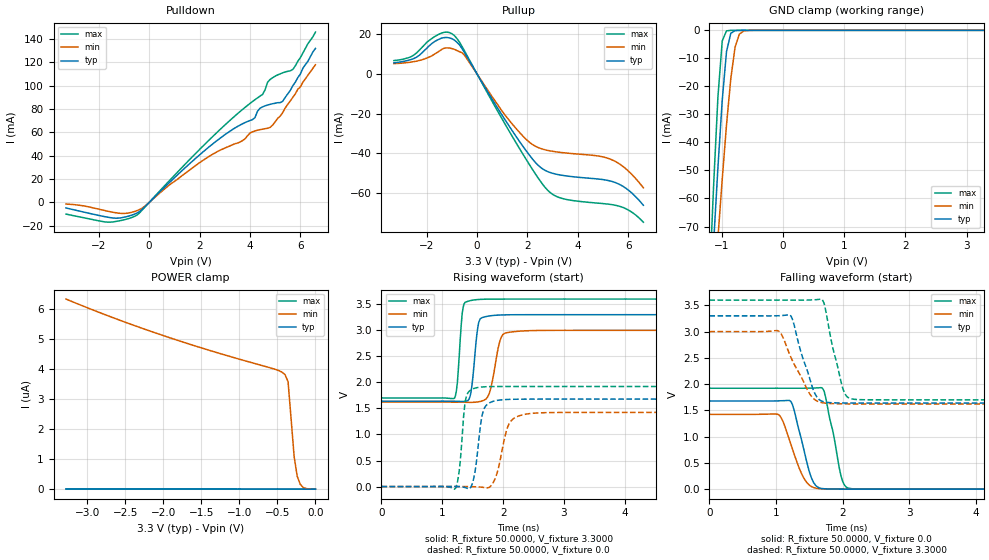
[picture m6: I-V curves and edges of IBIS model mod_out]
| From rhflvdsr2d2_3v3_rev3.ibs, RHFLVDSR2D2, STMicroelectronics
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|   Model mod_out
[Model]   mod_out
Model_type 3-state
Polarity   Non-Inverting
Enable   Active-High
Vmeas  =   1.650V
Cref   =   10pF
C_comp   0.640pF   0.584pF   0.702pF
[Temperature Range]  25.0000   0.1250k   -55.0000
[Voltage Range]   3.3000V   3.0000V   3.6000V
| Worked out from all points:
|   slope of the pulldown table from 0 to 0.495 V, typ, clamps not added: 46.8 ohm
|   slope of the pullup table from 0 to 0.495 V, typ, clamps not added: 46.9 ohm
|   GND clamp passes 1 mA (typ) near -0.85 V on its own axis
|   rising waveform, R_fixture 50.0000, V_fixture 3.3000: 20-80 % time 83.5ps typ, 133ps min, 66.4ps max; typ from 1.64 V to 3.3 V
|   rising waveform, R_fixture 50.0000, V_fixture 0.0: 20-80 % time 106ps typ, 167ps min, 81.1ps max; typ from 0 V to 1.68 V
|   falling waveform, R_fixture 50.0000, V_fixture 0.0: 20-80 % time 196ps typ, 239ps min, 176ps max; typ from 1.68 V to 0 V
|   falling waveform, R_fixture 50.0000, V_fixture 3.3000: 20-80 % time 236ps typ, 313ps min, 197ps max; typ from 3.3 V to 1.64 V
[Pulldown]
|Voltage   I(typ)   I(min)   I(max)
-3.3V     -4.744mA   -1.373mA   -9.997mA
-1.6V     -12.82mA   -7.695mA   -16.93mA
-1V       -12.69mA   -9.437mA   -14.89mA
-500mV    -9.257mA   -7.15mA    -11.05mA
2.4V      47.99mA    39.74mA    53.91mA
3.6V      66.23mA    51.68mA    77.75mA
4.1V      70.95mA    60.5mA     86.46mA
4.5V      81.9mA     62.8mA     92.56mA
4.8V      84.1mA     64.3mA     105.4mA
5.3V      86.7mA     77mA       111.1mA
5.7V      100mA      90mA       114mA
6.6V      132mA      118mA      146mA
[Pullup]
|Voltage   I(typ)   I(min)   I(max)
-3.3V     5.65mA     5.22mA     6.74mA
-2.4V     8.45mA     6.46mA     10.62mA
-1.5V     17.55mA    11.5mA     20.1mA
-1V       17.77mA    12.8mA     20.31mA
-500mV    10.83mA    9.442mA    11.64mA
1V        -20.88mA   -18.83mA   -22.78mA
1.8V      -36.04mA   -31mA      -39.95mA
2.8V      -49.13mA   -38.47mA   -58.51mA
3.5V      -51.26mA   -39.75mA   -63.05mA
5.3V      -53.92mA   -42.94mA   -65.68mA
5.9V      -57.48mA   -47.67mA   -67.81mA
6.6V      -66.12mA   -57.33mA   -74.62mA
[GND_clamp]
|Voltage   I(typ)   I(min)   I(max)
-3.3V     -1.037A    -847.3mA   -1.291A
-1.2V     -103.9mA   -118.4mA   -90.61mA
-1.13V    -75.7mA    -95.97mA   -55.15mA
-1.06V    -48.92mA   -74.09mA   -23.64mA
-990mV    -24.98mA   -53.14mA   -3.768mA
-920mV    -7.585mA   -33.75mA   -179.6uA
-850mV    -1.057mA   -17.22mA   -5.053uA
-780mV    -97.1uA    -5.969mA   -122.7nA
-710mV    -6.82uA    -1.339mA   -2.974nA
-640mV    -449.9nA   -233.7uA   -80.51pA
-500mV    -1.943nA   -4.459uA   -7.043pA
3.28V     3.538uA    1.987uA    6.819uA
[POWER_clamp]
|Voltage   I(typ)   I(min)   I(max)
-3.28V    10.31nA    6.317uA    198.2pA
-2.68V    8.946nA    5.716uA    177.1pA
-2.04V    7.686nA    5.138uA    154.7pA
-560mV    5.402nA    4.006uA    102.7pA
-440mV    5.247nA    3.889uA    98.42pA
-400mV    5.194nA    3.807uA    96.77pA
-360mV    5.137nA    3.571uA    94.08pA
-280mV    4.92nA     1.078uA    85.8pA
-240mV    4.209nA    433.6nA    68.63pA
-200mV    1.594nA    161nA      33.42pA
-160mV    407.8pA    56.33nA    25.64pA
0V        24.13pA    1.061nA    22.9pA
[Ramp]
| variable   typ   min   max
dV/dt_r  5.7510m/72.2785p   85.3302u/1.2075p   4.2267m/47.6152p
dV/dt_f  2.1600m/30.8571p   1.6200m/11.5166p   4.1400m/28.9055p
R_load = 50.0000
[Rising Waveform]
R_fixture= 50.0000
V_fixture= 3.3000
V_fixture_min= 3.0000
V_fixture_max= 3.6000
|time   V(typ)   V(min)   V(max)
0s        1.64V      1.621V     1.701V
1.2ns     1.639V     1.621V     1.695V
1.248ns   1.637V     1.62V      1.988V
1.328ns   1.633V     1.619V     3.327V
1.44ns    1.68V      1.617V     3.564V
1.584ns   3.05V      1.625V     3.591V
1.68ns    3.253V     1.655V     3.596V
1.952ns   3.294V     2.811V     3.6V
2.048ns   3.297V     2.951V     3.6V
6ns       3.3V       3V         3.6V
[Rising Waveform]
R_fixture= 50.0000
V_fixture= 0.0
V_fixture_min= 0.0
V_fixture_max= 0.0
|time   V(typ)   V(min)   V(max)
0s        69.89nV    38.92uV    8.651nV
1.224ns   1.324mV    451uV      -26.9mV
1.296ns   -3.189mV   620.2uV    483.1mV
1.376ns   -18.32mV   656.7uV    1.624V
1.536ns   267.9mV    -4.54mV    1.889V
1.664ns   1.408V     -14.11mV   1.913V
1.856ns   1.642V     118.1mV    1.92V
2.096ns   1.674V     1.198V     1.922V
2.336ns   1.678V     1.382V     1.922V
6ns       1.679V     1.424V     1.922V
[Falling Waveform]
R_fixture= 50.0000
V_fixture= 0.0
V_fixture_min= 0.0
V_fixture_max= 0.0
|time   V(typ)   V(min)   V(max)
0s        1.679V     1.424V     1.922V
1.028ns   1.681V     1.425V     1.922V
1.22ns    1.674V     870.1mV    1.922V
1.396ns   876.4mV    265.6mV    1.922V
1.532ns   216.9mV    49.44mV    1.925V
1.692ns   12.42mV    6.183mV    1.928V
1.748ns   6.091mV    3.735mV    1.736V
1.98ns    565.3uV    653.2uV    237.4mV
2.1ns     179.7uV    297.2uV    16.06mV
6ns       93.46nV    38.95uV    -27.31nV
[Falling Waveform]
R_fixture= 50.0000
V_fixture= 3.3000
V_fixture_min= 3.0000
V_fixture_max= 3.6000
|time   V(typ)   V(min)   V(max)
0s        3.3V       3V         3.6V
1.02ns    3.301V     3.019V     3.6V
1.212ns   3.312V     2.547V     3.6V
1.548ns   1.936V     1.745V     3.604V
1.692ns   1.674V     1.647V     3.611V
1.724ns   1.662V     1.641V     3.532V
1.852ns   1.645V     1.629V     2.697V
1.996ns   1.641V     1.624V     1.951V
2.124ns   1.64V      1.623V     1.723V
6ns       1.64V      1.621V     1.701V
